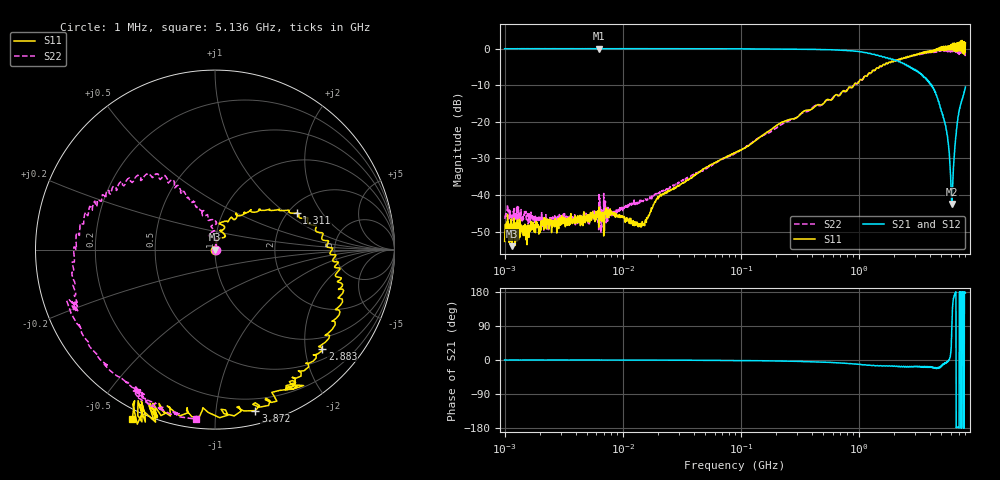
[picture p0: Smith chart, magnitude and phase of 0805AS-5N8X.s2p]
!s-Parameter Generated by FASTRON Sdn. Bhd.
!FASTRON P/N : 0805AS-5N8X
!Keysight Technologies: E5071C_MY46733604_B.14.02
!Date: Fri Nov 28 11:49:21 2025
!Version  :Rev01  Tue Jan 13 16:30:05 2026
!Data & Calibration Information:
!Freq  S11:SOLT2(ON)  S21:SOLT2(ON)  S12:SOLT2(ON)  S22:SOLT2(ON)
!PortZ  Port1:50+j0  Port2:50+j0
!When reading reference impedance value at option line is always used.
! Remarks : This data is being provided solely for informational purposes.
# Hz S dB R 50
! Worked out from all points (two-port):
!   1601 points, 1 MHz to 8 GHz, reference 50 ohm
!   highest |S21| = -0.01 dB at 6.301 MHz (marker M1); lowest = -42.5 dB at 6.149 GHz (marker M2)
!   |S21| within 3 dB of the highest: start of sweep to 1.962 GHz
!   lowest |S11| = -54.0 dB at 1.152 MHz (marker M3), VSWR 1.00, Z = 50.2 - j0.0602 ohm
!   |S11| at or under -10 dB: start of sweep to 909.3 MHz
!   |S22| runs from -50.4 to -0.3 dB; largest |S21 - S12| = 0.0081
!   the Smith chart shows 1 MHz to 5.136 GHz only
!   S11 on the Smith chart (normalised r, x): 1 MHz: 1.00, -0.00; 1.311 GHz: 2.23, +1.20; 2.883 GHz: 0.72, -2.37; 3.872 GHz: 0.10, -1.28; 5.136 GHz: -0.03, -0.62
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1000000  -52.70 -11.6  -0.05 -0.1  -0.04 -0.1  -46.50 5.0
1151819  -54.00 -17.5  -0.06 -0.1  -0.04 -0.0  -45.40 4.1
4479405  -47.10 16.4  -0.05 -0.1  -0.05 -0.1  -46.80 21.4
6301378  -43.30 28.0  -0.01 -0.4  -0.00 -0.1  -39.40 35.4
1.46648e7  -47.30 51.2  -0.04 -0.3  -0.06 -0.3  -41.70 42.6
2.00676e7  -40.60 54.2  -0.05 -0.3  -0.06 -0.3  -39.50 59.9
8.994653e7  -28.40 77.0  -0.07 -1.3  -0.08 -1.3  -28.60 79.1
4.006501e8  -16.50 80.2  -0.23 -4.6  -0.23 -4.6  -16.30 87.2
1.310879e9  -6.04 24.0  -1.58 -14.3  -1.59 -14.5  -6.05 124.0
1.7949e9  -3.78 0.9  -2.79 -15.6  -2.79 -15.9  -3.76 145.0
2.384191e9  -2.56 -17.2  -4.15 -17.0  -4.22 -17.3  -2.63 161.0
2.883048e9  -1.79 -42.7  -5.56 -16.7  -5.61 -16.6  -1.96 -174.0
3.872345e9  -0.68 -75.9  -8.72 -17.5  -8.72 -17.9  -1.08 -142.0
4.380627e9  -0.53 -109.0  -11.40 -21.7  -11.40 -22.1  -0.95 -117.0
4.828497e9  -0.03 -113.0  -15.30 -18.6  -15.30 -19.3  -0.72 -115.0
5.136407e9  0.43 -116.0  -18.00 -11.2  -18.10 -11.9  -0.46 -96.4
5.556285e9  0.35 -138.0  -22.70 -7.0  -22.70 -7.1  -0.47 -63.3
5.918038e9  0.78 -142.0  -31.20 7.0  -31.20 6.2  -0.67 -60.2
6.149367e9  0.59 -139.0  -42.50 91.3  -42.50 91.1  -0.35 -43.7
6.534915e9  1.30 -143.0  -26.40 177.0  -26.40 176.0  -0.31 -15.5
7.036128e9  0.67 -167.0  -17.30 -179.0  -17.40 -179.0  -0.79 13.4
8e9  1.61 157.0  -10.50 177.0  -10.40 177.0  -1.10 39.0
